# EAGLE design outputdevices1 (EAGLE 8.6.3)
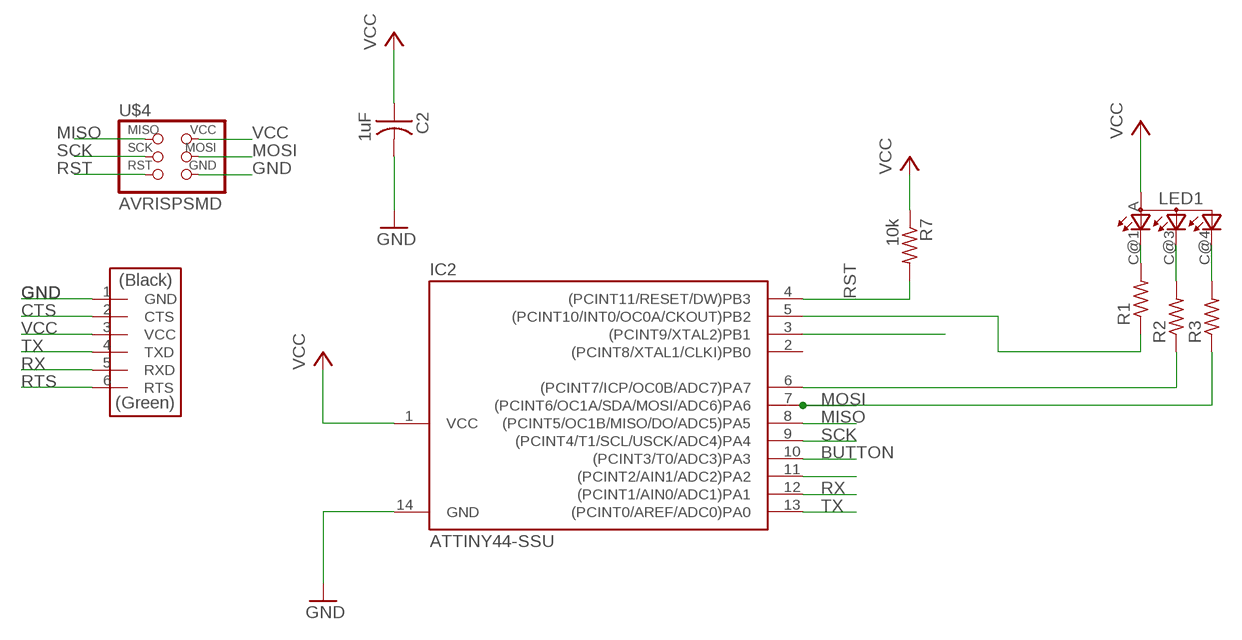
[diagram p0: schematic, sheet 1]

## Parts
C2  1uF  CAP-US1206  [C1206]
IC2  ATTINY44-SSU  [SOIC14]
LED1  TOPLED-3P-LCC-4  [P-LCC-4]
R1  RES-US1206FAB  [R1206FAB]
R2  RES-US1206FAB  [R1206FAB]
R3  RES-US1206FAB  [R1206FAB]
R7  10k  RES-US1206  [R1206]
U$4  AVRISPSMD  [2X03SMD]
U$6  FTDI-SMD-HEADER  [1X06SMD]

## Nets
BUTTON: IC2.10((PCINT3/T0/ADC3)PA3)
CTS: U$6.2(CTS)
GND: C2.2 IC2.14(GND) U$4.6(GND) U$6.1(GND)
MISO: IC2.8((PCINT5/OC1B/MISO/DO/ADC5)PA5) U$4.1(MISO)
MOSI: IC2.7((PCINT6/OC1A/SDA/MOSI/ADC6)PA6) R3.1 U$4.4(MOSI)
N$1: IC2.5((PCINT10/INT0/OC0A/CKOUT)PB2) R1.1
N$2: LED1.C@3(CBLUE) R2.2
N$3: LED1.C@4(CGREEN) R3.2
N$4: IC2.6((PCINT7/ICP/OC0B/ADC7)PA7) R2.1
N$5: LED1.C@1(CRED) R1.2
N$18: IC2.3((PCINT9/XTAL2)PB1)
N$24: IC2.11((PCINT2/AIN1/ADC2)PA2)
RST: IC2.4((PCINT11/RESET/DW)PB3) R7.2 U$4.5(RST)
RTS: U$6.6(RTS)
RX: IC2.12((PCINT1/AIN0/ADC1)PA1) U$6.5(RXD)
SCK: IC2.9((PCINT4/T1/SCL/USCK/ADC4)PA4) U$4.3(SCK)
TX: IC2.13((PCINT0/AREF/ADC0)PA0) U$6.4(TXD)
VCC: C2.1 IC2.1(VCC) LED1.A(A2) R7.1 U$4.2(VCC) U$6.3(VCC)
Unconnected: IC2.2((PCINT8/XTAL1/CLKI)PB0)

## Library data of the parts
C2 = fab:CAP-US
IC2 = fab:ATTINY44
LED1 = led:TOPLED-3: OSRAM - Hyper Multi TOPLED® (RGB) LB E673, LV E673, LT E673 - Power TOPLED® Enhanced optical Power LED (HOP2000) LS E67B, LA E67B, LO E67B, LY E67B - Hyper Multi TOPLED® Enhanced optical Power LED (HOP2000 / ATON®) LATB T66B - Hyper Multi TOPLED® Hyper-Bright LED LATB T686 Source: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
R1-R3 R7 = fab:RES-US: Resistor (US Symbol)
U$4 = fab:AVRISP
U$6 = fab:FTDI-SMD-HEADER

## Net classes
0 default: width 0.03 mm, drill 0.051 mm, clearance 0.025 mm

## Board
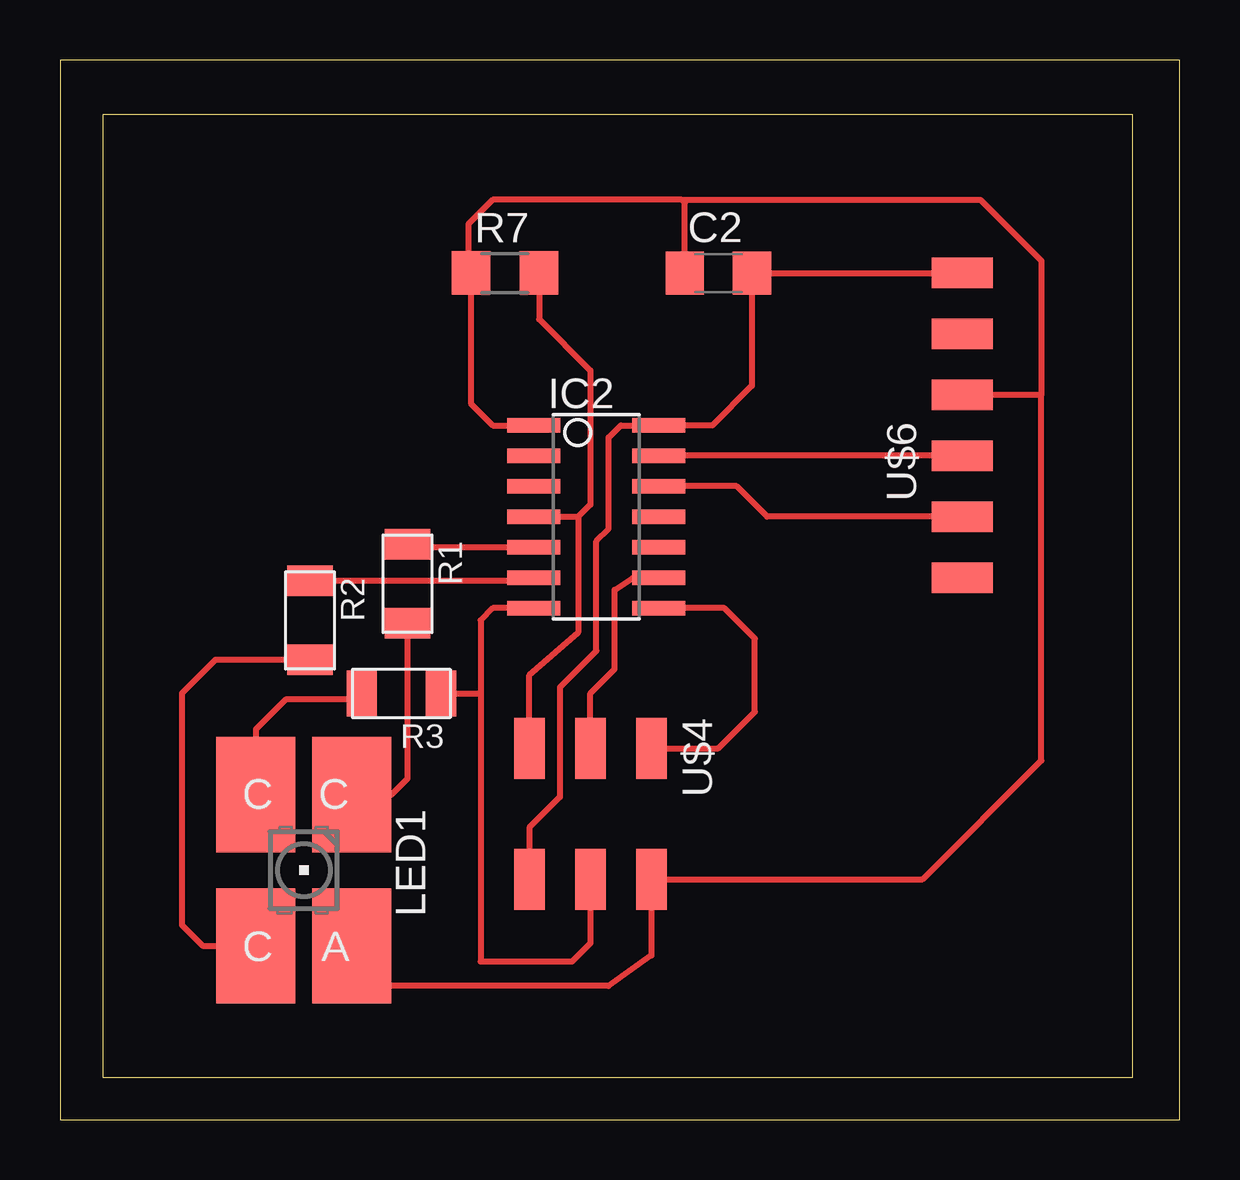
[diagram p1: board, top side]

Size 46.66 x 44.19 mm. Coordinates in mm from the lower left corner, seen from the top.
Outline: 0,0 46.66,0 46.66,44.19 0,44.19 0,0
Copper layers (1*16): Top 0.035mm / dielectric 1.5mm / Bottom 0.035mm
Design rules "default": minimum track width 6mil, minimum drill 0.35mm, track to track 6mil, track to pad 6mil, pad to pad 6mil, via to via 6mil, smd to smd 6mil, copper to edge 40mil, drill to drill 6mil, minimum pad ring 10mil, minimum via ring 8mil, stop-mask expansion 4mil, vias tented up to drill 0mil, thermal gap 10mil
Milling: area 1.8,1.8 to 44.7,41.9

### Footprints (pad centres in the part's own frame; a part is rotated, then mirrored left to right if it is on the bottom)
C1206 = smd 1.6 x 1.8: 1 -1.4,0; 2 1.4,0
SOIC14 = smd 0.61 x 2.21: 1 -3.81,-2.603; 2 -2.54,-2.603; 3 -1.27,-2.603; 4 0,-2.603; 5 1.27,-2.603; 6 2.54,-2.603; 7 3.81,-2.603; 8 3.81,2.603; 9 2.54,2.603; 10 1.27,2.603; 11 0,2.603; 12 -1.27,2.603; 13 -2.54,2.603; 14 -3.81,2.603
P-LCC-4 = smd 3.3 x 4.8: A -2,3.15; C@1 -2,-3.15; C@3 2,3.15; C@4 2,-3.15
R1206FAB = smd 1.27 x 1.905: 1 -1.651,0; 2 1.651,0
R1206 = smd 1.6 x 1.803: 1 -1.422,0; 2 1.422,0
2X03SMD = smd 2.54 x 1.27: 1 -2.54,2.54; 2 2.92,2.54; 3 -2.54,0; 4 2.92,0; 5 -2.54,-2.54; 6 2.92,-2.54
1X06SMD = smd 2.54 x 1.27: 1 0,6.35; 2 0,3.81; 3 0,1.27; 4 0,-1.27; 5 0,-3.81; 6 0,-6.35

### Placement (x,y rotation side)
C2  27.43,35.31 0 top
IC2  22.35,25.15 270 top
LED1  10.16,10.41 180 top
R1  14.48,22.35 270 top
R2  10.41,20.83 270 top
R3  14.22,17.78 180 top
R7  18.54,35.31 0 top
U$4  22.1,12.95 270 top
U$6  37.59,28.96 0 top

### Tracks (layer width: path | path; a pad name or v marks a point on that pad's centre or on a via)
GND
  Top 0.254: U$6.1 C2.2 28.83,30.61 27.18,28.96 IC2.14 23.37,28.96 22.86,28.45 22.86,24.64 22.35,24.13 22.35,19.56 20.83,18.03 20.83,13.46 19.56,12.19 U$4.6
MISO
  Top 0.254: U$4.1 27.43,15.49 28.96,17.02 28.96,20.07 27.69,21.34 IC2.8
MOSI
  Top 0.254: U$4.4 22.1,7.37 21.34,6.6 17.53,6.6 17.53,17.78 | IC2.7 18.03,21.34 17.53,20.83 17.53,17.78 | R3.1 17.53,17.78
N$1
  Top 0.254: R1.1 14.61,23.88 IC2.5
N$2
  Top 0.254: R2.2 6.48,19.18 5.08,17.78 5.08,8.13 5.94,7.26 LED1.C@3
N$3
  Top 0.254: R3.2 12.32,17.53 9.4,17.53 8.16,16.29 LED1.C@4
N$4
  Top 0.254: R2.1 19.62,22.48 IC2.6
N$5
  Top 0.254: R1.2 14.48,14.22 13.82,13.56 LED1.C@1
RST
  Top 0.254: 21.59,25.15 21.59,20.32 19.56,18.54 U$4.5 | IC2.4 21.59,25.15 | 21.59,25.15 22.1,25.65 22.1,31.24 19.96,33.38 R7.2
RX
  Top 0.254: IC2.12 28.19,26.42 29.46,25.15 U$6.5
SCK
  Top 0.254: U$4.3 22.1,17.78 23.11,18.8 23.11,22.1 23.88,22.61 IC2.9
TX
  Top 0.254: U$6.4 IC2.13
VCC
  Top 0.254: IC2.1 18.03,28.96 17.12,29.87 R7.1 17.02,35.41 17.02,37.34 18.03,38.35 25.91,38.35 | C2.1 26.03,38.23 25.91,38.35 | 25.91,38.35 38.35,38.35 40.89,35.81 40.89,30.23 | 40.89,30.23 U$6.3 | 40.89,30.23 40.89,14.99 35.94,10.03 U$4.2 24.64,6.86 22.86,5.59 12.45,5.59 12.16,5.87 LED1.A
